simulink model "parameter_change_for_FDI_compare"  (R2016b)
settings: Solver=ode45  StartTime=0.0  StopTime=1020  RelTol=1e-3  EnableMultiTasking=on
libraries: ctrlSharedLib x1

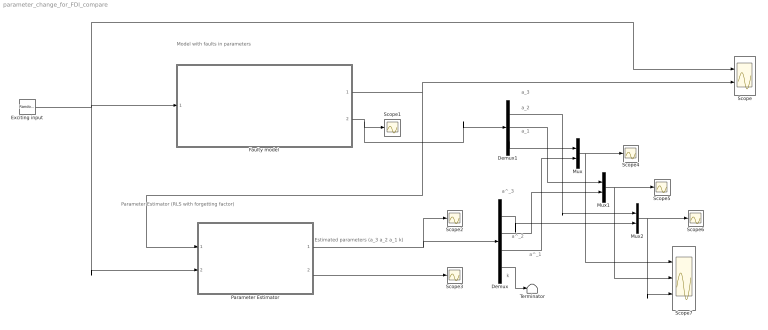
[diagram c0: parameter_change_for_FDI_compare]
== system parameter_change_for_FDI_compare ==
  note: k
  note: Estimated parameters (a_3 a_2 a_1 k)
  note: a_1
  note: a_2
  note: a_3
  note: Parameter Estimator (RLS with forgetting factor)
  note: Model with faults in parameters
  note: a^_3
  note: a^_2
  note: a^_1
  Demux : Demux
  Demux1 : Demux  Outputs=3
  Exciting input : RandomNumber  Variance=0.4/(0.6388)^2  Seed=1  SampleTime=1
  Faulty model : Subsystem
  Mux : Mux  Inputs=2
  Mux1 : Mux  Inputs=2
  Mux2 : Mux  Inputs=2
  Parameter Estimator : Subsystem
  Scope : Scope  NumInputPorts=2
  Scope{1..6} (6 alike) : Scope
  Scope7 : Scope  NumInputPorts=3
  Terminator : Terminator
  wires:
  Demux/2 -> Mux1/2
  Demux/4 -> Terminator/1
  Faulty model/1(y(t)) -> Parameter Estimator/1(y(t)), Scope/2
  Parameter Estimator/1(Parameters) -> Scope2/1, Demux/1
  Parameter Estimator/2(Error) -> Scope3/1
  Exciting input/1 -> Parameter Estimator/2(u(t)), Faulty model/1(u*(t)), Scope/1
  Faulty model/2(\Theta) -> Demux1/1, Scope1/1
  Demux1/3 -> Mux/1
  Mux/1 -> Scope7/1, Scope4/1
  Mux1/1 -> Scope7/2, Scope5/1
  Mux2/1 -> Scope7/3, Scope6/1
  Demux1/2 -> Mux1/1
  Demux1/1 -> Mux2/1
  Demux/3 -> Mux/2
  Demux/1 -> Mux2/2

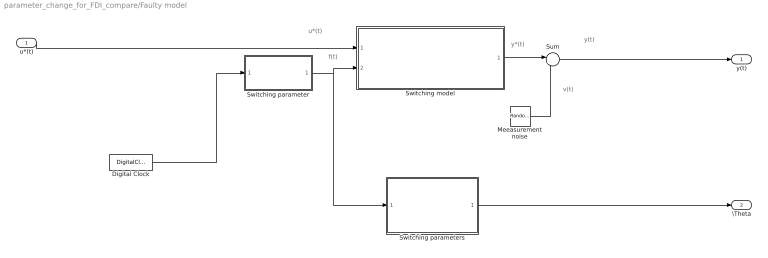
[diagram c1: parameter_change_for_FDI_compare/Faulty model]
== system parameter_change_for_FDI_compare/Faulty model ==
  note: u*(t)
  note: y(t)
  note: y*(t)
  note: v(t)
  note: f(t)
  u*(t) : Inport
  Digital Clock : DigitalClock
  Meeasurement noise : RandomNumber  Variance=(0.01)^2  Seed=3  SampleTime=1
  Sum : Sum  Inputs=|++  SaturateOnIntegerOverflow=on
  Switching parameter : Subsystem
  Switching model : Subsystem
  Switching parameters : Subsystem
  y(t) : Outport
  \Theta : Outport  Port=2
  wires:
  Sum/1 -> y(t)/1
  Switching parameter/1(a(t)) -> Switching parameters/1(f(t)), Switching model/2(f(t))
  Switching model/1(y*(t)) -> Sum/1
  u*(t)/1 -> Switching model/1(u*(t))
  Meeasurement noise/1 -> Sum/2
  Digital Clock/1 -> Switching parameter/1(t)
  Switching parameters/1(\Theta) -> \Theta/1

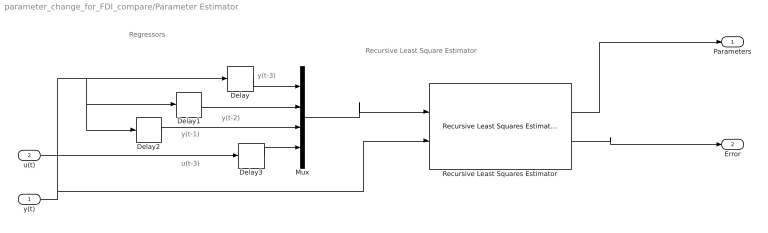
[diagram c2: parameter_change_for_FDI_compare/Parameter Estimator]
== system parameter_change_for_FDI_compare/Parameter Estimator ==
  note: Regressors
  note: Recursive Least Square Estimator
  note: y(t-3)
  note: y(t-2)
  note: y(t-1)
  note: u(t-3)
  y(t) : Inport
  u(t) : Inport  Port=2
  Delay : Delay  DelayLength=3  SampleTime=1
  Delay1 : Delay  SampleTime=1
  Delay2 : Delay  DelayLength=1  SampleTime=1
  Delay3 : Delay  DelayLength=3  SampleTime=1
  Mux : Mux
  Recursive Least Squares Estimator : ctrlSharedLib/Recursive Least Squares Estimator  InitialEstimateSource=None  InitialParameterData=4  P0=1e4  InitialRegressors=0  InitialOutputs=0  History=Infinite  WindowLength=200  EstimationMethod=Forgetting Factor  AdaptationParameter=lambda  HasTimeVaryingAdaptationParameter=off  NormalizationBias=eps  OutputError=on  OutputP=off  AddEnablePort=off  InputProcessing=Sample-based  Ts=1
  Parameters : Outport
  Error : Outport  Port=2
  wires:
  y(t)/1 -> Delay1/1, Delay2/1, Delay/1, Recursive Least Squares Estimator/2
  Recursive Least Squares Estimator/2 -> Error/1
  Delay/1 -> Mux/1
  Delay2/1 -> Mux/3
  Recursive Least Squares Estimator/1 -> Parameters/1
  Mux/1 -> Recursive Least Squares Estimator/1
  Delay3/1 -> Mux/4
  Delay1/1 -> Mux/2
  u(t)/1 -> Delay3/1

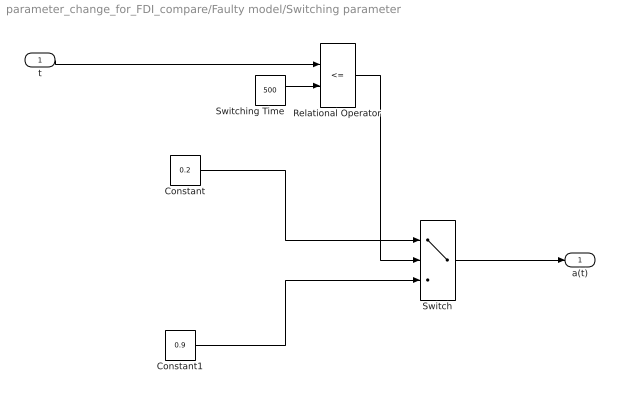
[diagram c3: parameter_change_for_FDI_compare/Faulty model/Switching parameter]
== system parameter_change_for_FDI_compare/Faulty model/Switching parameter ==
  t : Inport
  Constant : Constant  Value=0.2
  Constant1 : Constant  Value=0.9
  Relational Operator : RelationalOperator  Operator=<=
  Switch : Switch  Threshold=1
  Switching Time : Constant  Value=500
  a(t) : Outport
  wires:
  Constant/1 -> Switch/1
  Constant1/1 -> Switch/3
  Switching Time/1 -> Relational Operator/2
  Relational Operator/1 -> Switch/2
  Switch/1 -> a(t)/1
  t/1 -> Relational Operator/1

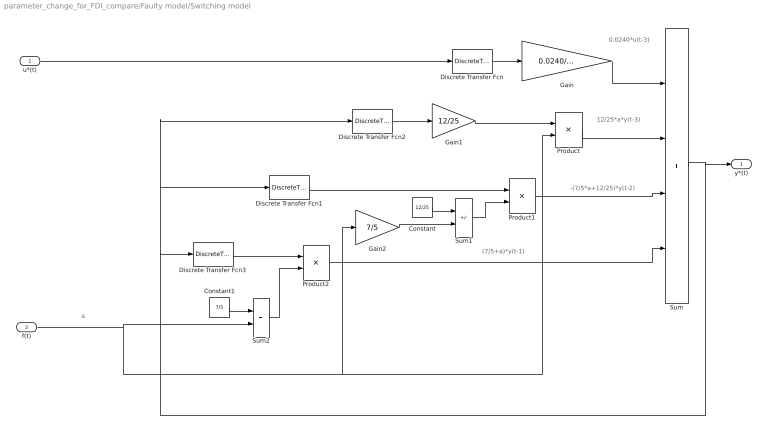
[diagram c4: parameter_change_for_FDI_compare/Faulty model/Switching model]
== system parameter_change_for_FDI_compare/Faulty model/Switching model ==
  note: 0.0240*u(t-3)
  note: 12/25*a*y(t-3)
  note: -(7/5*a+12/25)*y(t-2)
  note: a
  note: (7/5+a)*y(t-1)
  u*(t) : Inport
  f(t) : Inport  Port=2
  Constant : Constant  Value=12/25
  Constant1 : Constant  Value=7/5
  Discrete Transfer Fcn : DiscreteTransferFcn  Denominator=[1 0 0 0]  SampleTime=1
  Discrete Transfer Fcn1 : DiscreteTransferFcn  Denominator=[1 0 0]  SampleTime=1
  Discrete Transfer Fcn2 : DiscreteTransferFcn  Denominator=[1 0 0 0]  SampleTime=1
  Discrete Transfer Fcn3 : DiscreteTransferFcn  Denominator=[1 0]  SampleTime=1
  Gain : Gain  Gain=0.0240/0.1304  SaturateOnIntegerOverflow=on
  Gain1 : Gain  Gain=12/25  SaturateOnIntegerOverflow=on
  Gain2 : Gain  Gain=7/5  SaturateOnIntegerOverflow=on
  Product : Product  SaturateOnIntegerOverflow=on
  Product1 : Product  SaturateOnIntegerOverflow=on
  Product2 : Product  SaturateOnIntegerOverflow=on
  Sum : Sum  Inputs=++++  SaturateOnIntegerOverflow=on
  Sum1 : Sum  Inputs=--  SaturateOnIntegerOverflow=on
  Sum2 : Sum  SaturateOnIntegerOverflow=on
  y*(t) : Outport
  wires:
  Discrete Transfer Fcn/1 -> Gain/1
  Sum/1 -> y*(t)/1, Discrete Transfer Fcn2/1, Discrete Transfer Fcn1/1, Discrete Transfer Fcn3/1
  Gain/1 -> Sum/1
  u*(t)/1 -> Discrete Transfer Fcn/1
  Discrete Transfer Fcn2/1 -> Gain1/1
  Product/1 -> Sum/2
  Gain1/1 -> Product/1
  Product1/1 -> Sum/3
  Discrete Transfer Fcn1/1 -> Product1/1
  Gain2/1 -> Sum1/2
  Sum1/1 -> Product1/2
  Constant/1 -> Sum1/1
  f(t)/1 -> Sum2/2, Gain2/1, Product/2
  Product2/1 -> Sum/4
  Discrete Transfer Fcn3/1 -> Product2/1
  Constant1/1 -> Sum2/1
  Sum2/1 -> Product2/2

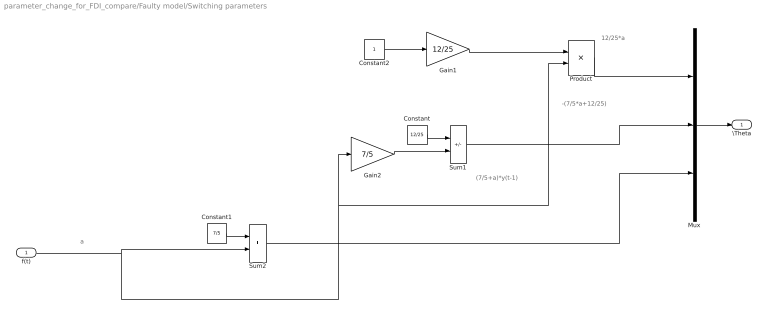
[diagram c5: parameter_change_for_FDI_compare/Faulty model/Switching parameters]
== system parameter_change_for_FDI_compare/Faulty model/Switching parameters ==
  note: (7/5+a)*y(t-1)
  note: -(7/5*a+12/25)
  note: a
  note: 12/25*a
  f(t) : Inport
  Constant : Constant  Value=12/25
  Constant1 : Constant  Value=7/5
  Constant2 : Constant
  Gain1 : Gain  Gain=12/25  SaturateOnIntegerOverflow=on
  Gain2 : Gain  Gain=7/5  SaturateOnIntegerOverflow=on
  Mux : Mux  Inputs=3
  Product : Product  SaturateOnIntegerOverflow=on
  Sum1 : Sum  Inputs=--  SaturateOnIntegerOverflow=on
  Sum2 : Sum  SaturateOnIntegerOverflow=on
  \Theta : Outport
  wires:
  Product/1 -> Mux/1
  Constant1/1 -> Sum2/1
  Constant2/1 -> Gain1/1
  Sum2/1 -> Mux/3
  Constant/1 -> Sum1/1
  f(t)/1 -> Sum2/2, Gain2/1, Product/2
  Gain2/1 -> Sum1/2
  Sum1/1 -> Mux/2
  Gain1/1 -> Product/1
  Mux/1 -> \Theta/1
